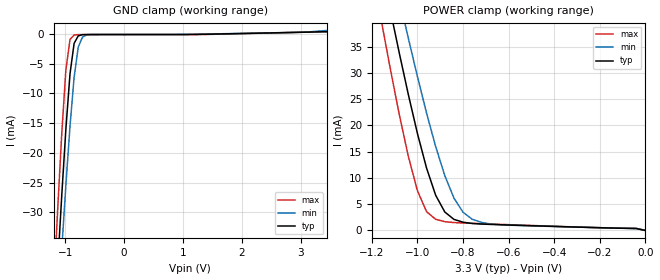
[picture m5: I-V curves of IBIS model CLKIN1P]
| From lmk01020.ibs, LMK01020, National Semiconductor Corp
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|   Model CLKIN1P
[Model]  CLKIN1P
Model_type Input
Polarity   Non-Inverting
Vinl =   1.5300V
Vinh =   1.7300V
C_comp   1.151pF   1.151pF   1.151pF
[Temperature Range]   25.0000   85.0000   -40.0000
[Voltage Range]   3.3000V   3.1500V   3.4500V
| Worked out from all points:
|   GND clamp passes 1 mA (typ) near -0.82 V on its own axis
|   POWER clamp passes 1 mA (typ) near -0.57 V on its own axis
[GND_clamp]
|Voltage   I(typ)   I(min)   I(max)
-3.45V    -488.6mA   -451mA     -506.6mA
-1.2V     -51.66mA   -58.95mA   -43.37mA
-1.13V    -39.16mA   -47.42mA   -29.63mA
-1.06V    -27.13mA   -36.19mA   -16.75mA
-990mV    -15.98mA   -25.44mA   -6.053mA
-920mV    -6.721mA   -15.53mA   -930.4uA
-850mV    -1.576mA   -7.276mA   -176.4uA
-780mV    -328.7uA   -2.224mA   -115.1uA
-710mV    -121.2uA   -560.8uA   -112.7uA
-640mV    -99.89uA   -172.9uA   -112.6uA
2.3V      134.7uA    149.3uA    118.3uA
3.45V     380.2uA    588uA      374uA
[POWER_clamp]
|Voltage   I(typ)   I(min)   I(max)
-3.45V    578.6mA    549mA      626.7mA
-1.16V    50.67mA    59.87mA    40.27mA
-1.12V    42.13mA    51.94mA    30.97mA
-1.08V    33.82mA    44.16mA    22.13mA
-1.04V    25.86mA    36.58mA    14.09mA
-1V       18.44mA    29.27mA    7.547mA
-960mV    11.86mA    22.33mA    3.579mA
-920mV    6.689mA    15.96mA    2.119mA
-880mV    3.513mA    10.43mA    1.67mA
-800mV    1.572mA    3.473mA    1.423mA
-680mV    1.155mA    1.25mA     1.23mA
0V        350.2pA    342.7pA    390.5pA
